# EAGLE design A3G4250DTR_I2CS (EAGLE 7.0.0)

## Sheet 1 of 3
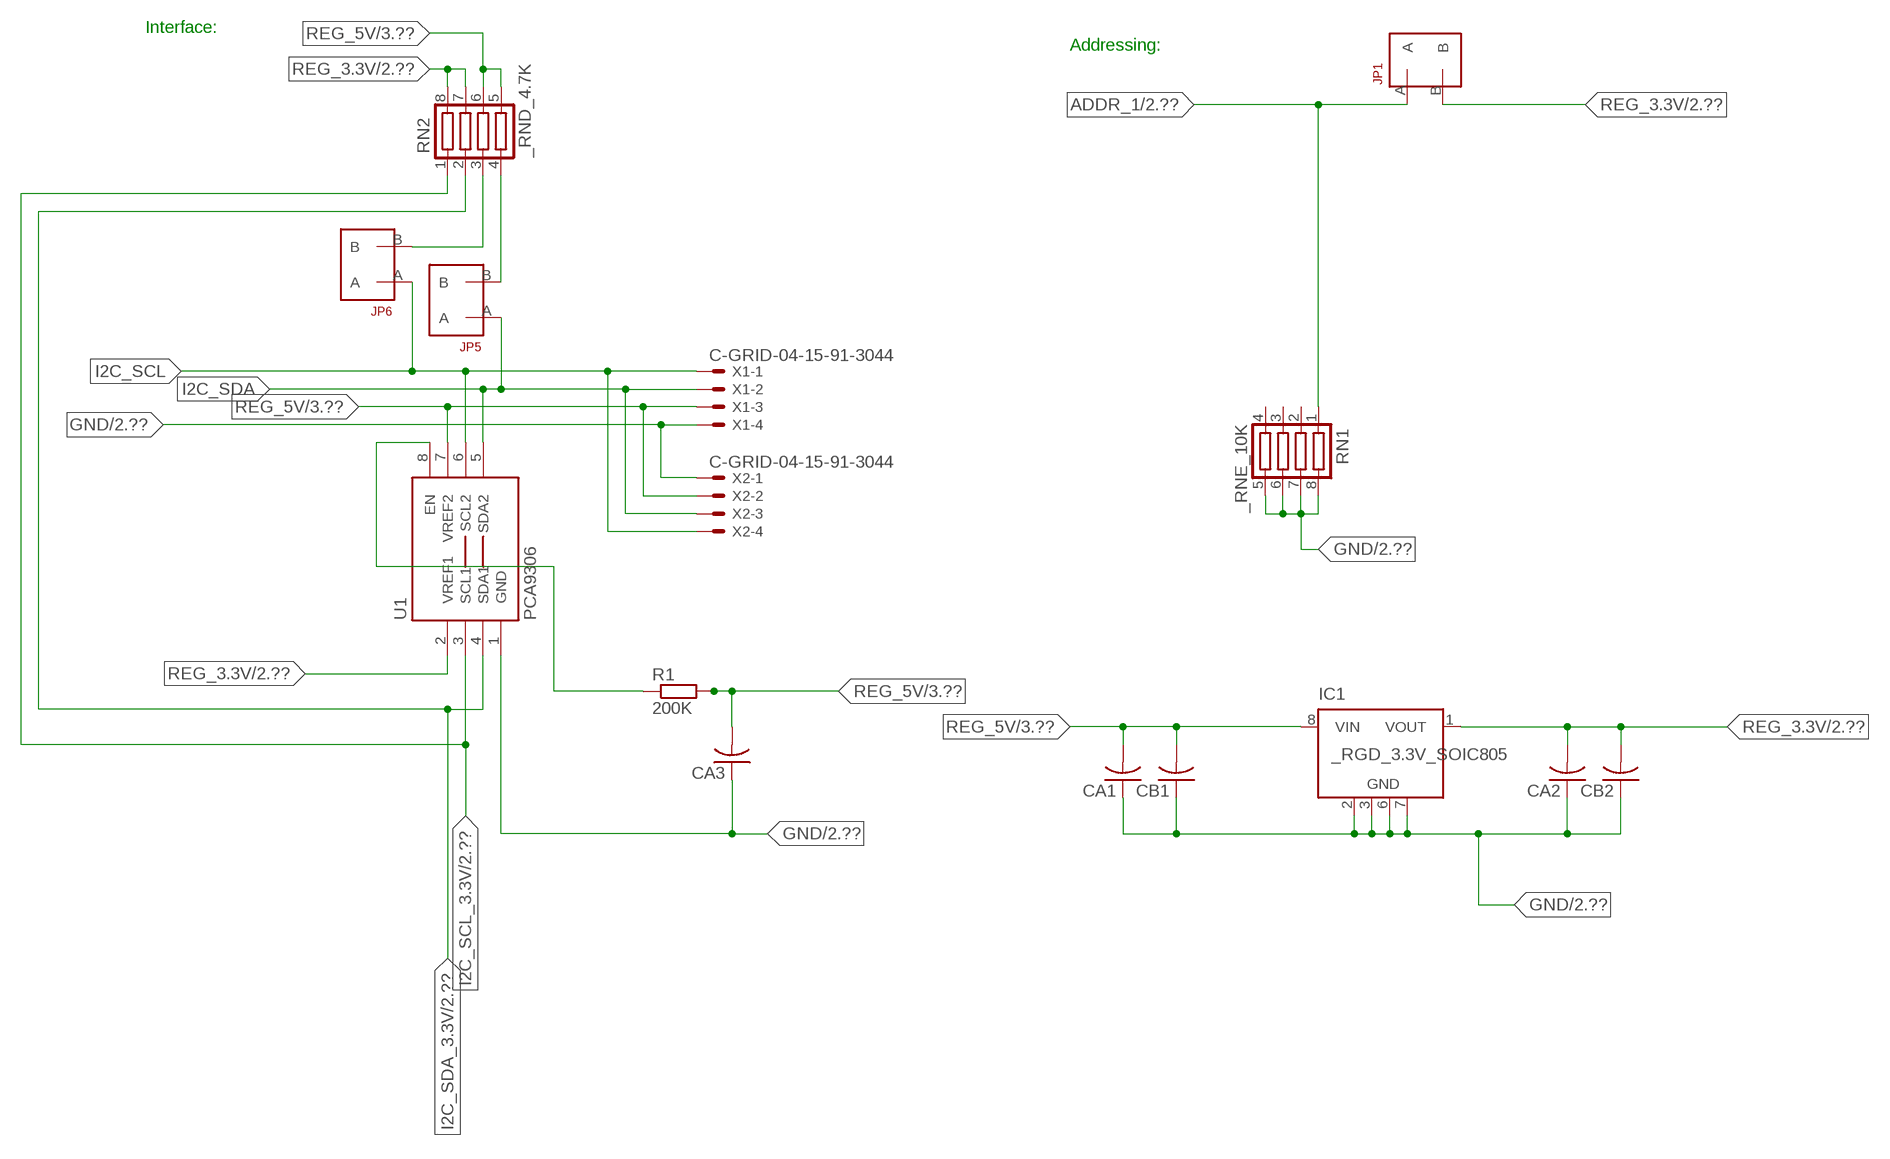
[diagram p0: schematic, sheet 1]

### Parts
CA1  CC1206KRX7R9BB104  [.1UF]
CA2  CC1206KRX7R9BB104  [.1UF]
CA3  CC1206KRX7R9BB104  [.1UF]
CB1  TMK316F106ZL-TC1206K  [TMK316F106ZL-T]
CB2  TMK316F106ZL-TC1206K  [TMK316F106ZL-T]
IC1  _RGD_3.3V_SOIC805  [_RGC_3.3V_SOIC8]
JP1  JUMPER_1X2_2MM  [JUMPER_1X2_2MM]
JP5  JUMPER_1X2_2MM  [JUMPER_1X2_2MM]
JP6  JUMPER_1X2_2MM  [JUMPER_1X2_2MM]
R1  200K  RESISTOR_SMT-0603  [R603]
RN1  _RNE_10K  [RNE]
RN2  _RND_4.7K  [RND]
U1  PCA9306  PCA9306_NCD  [PSOP-8]
X1  C-GRID-04-15-91-3044  [15-91-04]
X2  C-GRID-04-15-91-3044  [15-91-04]

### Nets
ADDR_1: JP1.A RN1.1 ; also sheet 2
GND: CA1.1 CA2.1 CA3.1 CB1.1 CB2.1 IC1.2(GND) IC1.3(GND) IC1.6(GND) IC1.7(GND) RN1.5 RN1.6 RN1.7 RN1.8 U1.1(GND) X1.4 X2.1 ; also sheet 2,3
I2C_SCL: JP6.A U1.6(SCL2) X1.1 X2.4
I2C_SCL_3.3V: RN2.1 U1.3(SCL1) ; also sheet 2
I2C_SDA: JP5.A U1.5(SDA2) X1.2 X2.3
I2C_SDA_3.3V: RN2.2 U1.4(SDA1) ; also sheet 2
N$1: JP6.B RN2.3
N$2: JP5.B RN2.4
N$3: R1.1 U1.8(EN)
REG_3.3V: CA2.2 CB2.2 IC1.1(VOUT) JP1.B RN2.7 RN2.8 U1.2(VREF1) ; also sheet 2
REG_5V: CA1.2 CA3.2 CB1.2 IC1.8(VIN) R1.2 RN2.5 RN2.6 U1.7(VREF2) X1.3 X2.2 ; also sheet 3
Unconnected: IC1.4(NC) IC1.5(NC) RN1.2 RN1.3 RN1.4

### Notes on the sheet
- Interface:
- Addressing:

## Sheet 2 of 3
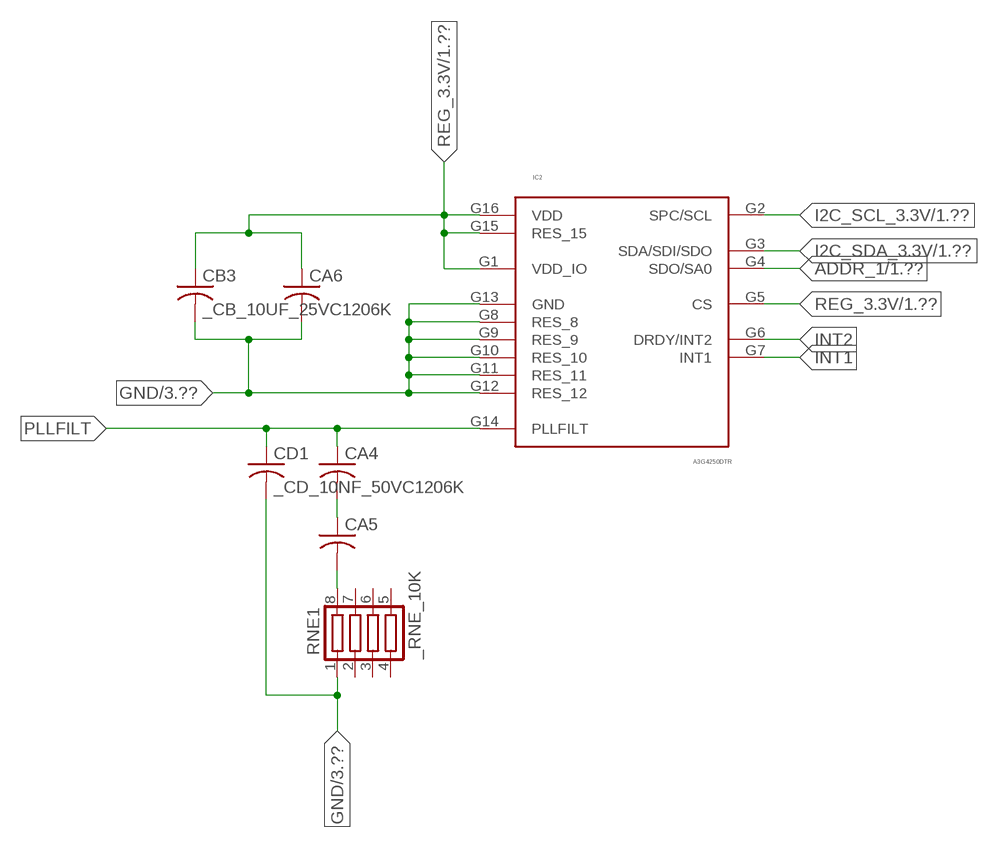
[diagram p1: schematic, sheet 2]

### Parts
CA4  _CA_.10UF_50VC1206K  [_CA_.1UF_50V]
CA5  _CA_.10UF_50VC1206K  [_CA_.1UF_50V]
CA6  _CA_.10UF_50VC1206K  [_CA_.1UF_50V]
CB3  _CB_10UF_25VC1206K  [_CB_10UF_25V]
CD1  _CD_10NF_50VC1206K  [_CD_10NF_50V]
IC2  A3G4250DTR  A3G4250D  [LGA-16]
RNE1  _RNE_10K  [RNE]

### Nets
ADDR_1: IC2.G4(SDO/SA0) ; also sheet 1
GND: CA6.2 CB3.2 CD1.2 IC2.G8(RES_8) IC2.G9(RES_9) IC2.G10(RES_10) IC2.G11(RES_11) IC2.G12(RES_12) IC2.G13(GND) RNE1.1 ; also sheet 1,3
I2C_SCL_3.3V: IC2.G2(SPC/SCL) ; also sheet 1
I2C_SDA_3.3V: IC2.G3(SDA/SDI/SDO) ; also sheet 1
INT1: IC2.G7(INT1)
INT2: IC2.G6(DRDY/INT2)
N$23: CA5.2 RNE1.8
N$24: CA4.2 CA5.1
PLLFILT: CA4.1 CD1.1 IC2.G14(PLLFILT)
REG_3.3V: CA6.1 CB3.1 IC2.G1(VDD_IO) IC2.G5(CS) IC2.G15(RES_15) IC2.G16(VDD) ; also sheet 1
Unconnected: RNE1.2 RNE1.3 RNE1.4 RNE1.5 RNE1.6 RNE1.7

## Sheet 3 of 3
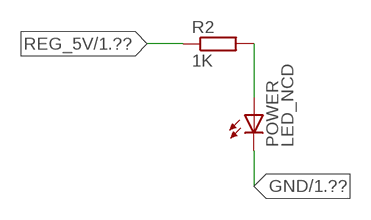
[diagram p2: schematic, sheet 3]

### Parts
POWER  LED_NCD  [CHIPLED_0603]
R2  1K  RESISTOR_SMT-0402  [R402]

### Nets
GND: POWER.C ; also sheet 1,2
N$4: POWER.A R2.2
REG_5V: R2.1 ; also sheet 1

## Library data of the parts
CA1-CA3 = NCD_ULTIMATE_LIBRARY:CC1206KRX7R9BB104: Capacitor CA .1uF 50V SMT C1206K CC1206KRX7R9BB104
CA4-CA6 = NCD_ULTIMATE_LIBRARY (2):_CA_.10UF_50V: Capacitor .1uF SMT
CB1 CB2 = NCD_ULTIMATE_LIBRARY:TMK316F106ZL-T: Capacitor CB 10uF SMT 1206 TMK316F106ZL-T
CB3 = NCD_ULTIMATE_LIBRARY (2):_CB_10UF_25V: Capacitor 10uF SMT
CD1 = NCD_ULTIMATE_LIBRARY (2):_CD_10NF_50V: Capacitor 10nF SMT
IC1 = NCD_ULTIMATE_LIBRARY:_RGD_3.3V_SOIC8: Regulator Linear 3.3V Chip Positive VOLTAGE REGULATOR Digikey 497-1199-2-ND/L78L33ACD13TR
IC2 = NCD_ULTIMATE_KAMNA:A3G4250D
JP1 JP5 JP6 = NCD_ULTIMATE_CONNECTORS:JUMPER_1X2_2MM
POWER = NCD_ULTIMATE_LIBRARY:LED_NCD: LED Digikey 754-1132-2-ND/APT2012SRCPRV
R1 R2 = NCD_ULTIMATE_LIBRARY:RESISTOR_SMT: NCD Resistor
RN1 = NCD_ULTIMATE_LIBRARY:_RNE_10K: Resistor Array RNE SMT 10K x 4 Single Resistor Source: http://www.ctscorp.com/components/Datasheets/CTSChipArrayDs.pdf Digikey 742C083103JPTR-ND/742C083103JP; OC_FARNELL: unknown; OC_NEWARK: unknown
RN2 = NCD_ULTIMATE_LIBRARY:_RND_4.7K: Resistor Array RND SMT 4.7K x 4 Single Resistor Source: http://www.ctscorp.com/components/Datasheets/CTSChipArrayDs.pdf Digikey 742C083472JPTR-ND/742C083472JP; OC_FARNELL: unknown; OC_NEWARK: unknown
RNE1 = NCD_ULTIMATE_LIBRARY (2):_RNE_10K: Resistor Array RNE SMT 10K x 4 Single Resistor Source: http://www.ctscorp.com/components/Datasheets/CTSChipArrayDs.pdf Digikey 742C083103JPTR-ND/742C083103JP; OC_FARNELL: unknown; OC_NEWARK: unknown
U1 = NCD_ULTIMATE_LIBRARY:PCA9306_NCD: NCD Bidirectional I2C level shifter. NOT compatible with all available part number pinout schemes- DOUBLE CHECK!!!; PROD_ID: IC-10023
X1 X2 = NCD_ULTIMATE_CONNECTORS:C-GRID-04: CONNECTOR 4-Pos I2C wire to board 2.54 mm (0.100") pitch header Digikey WM1342-ND/0015912045; OC_FARNELL: unknown; OC_NEWARK: unknown

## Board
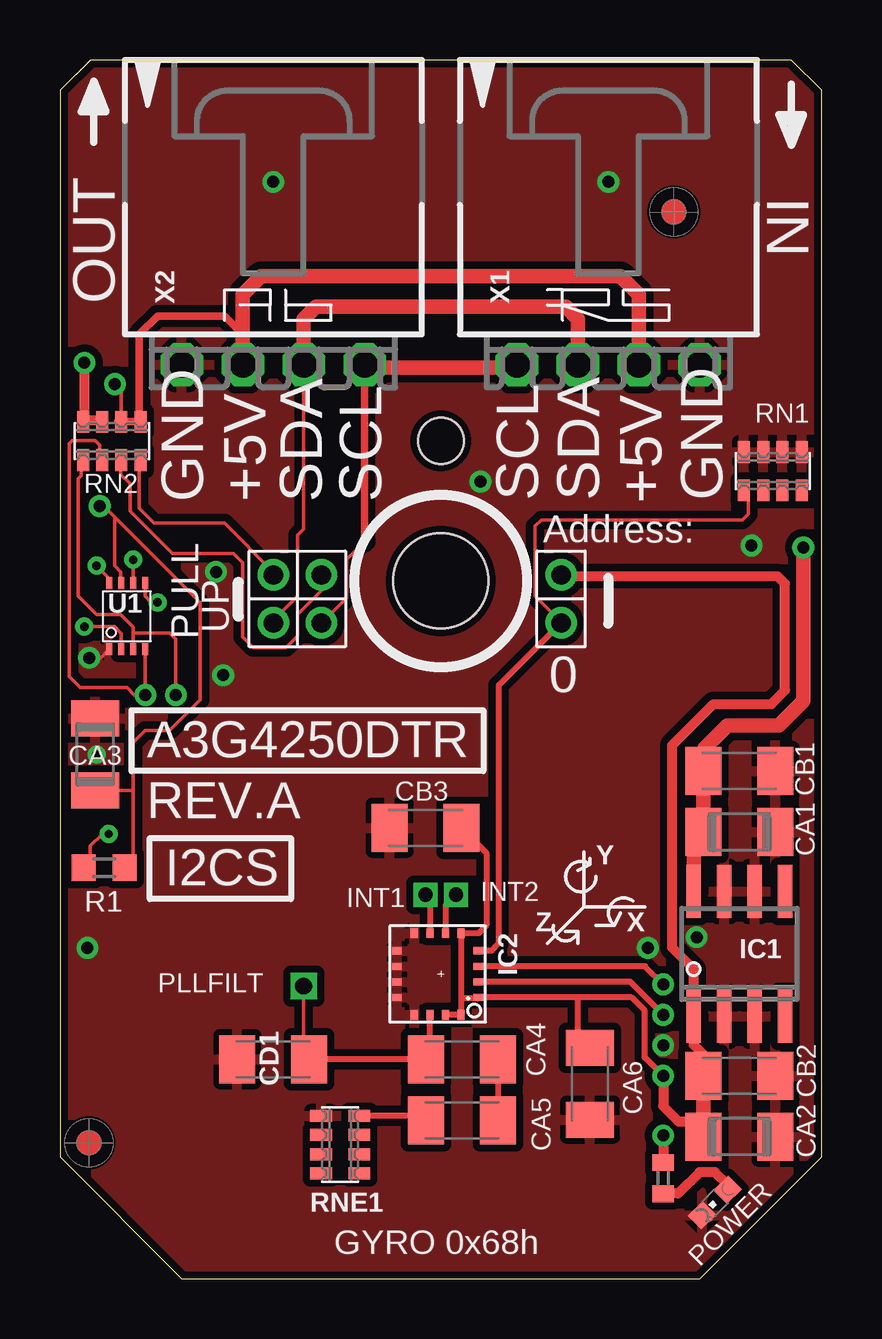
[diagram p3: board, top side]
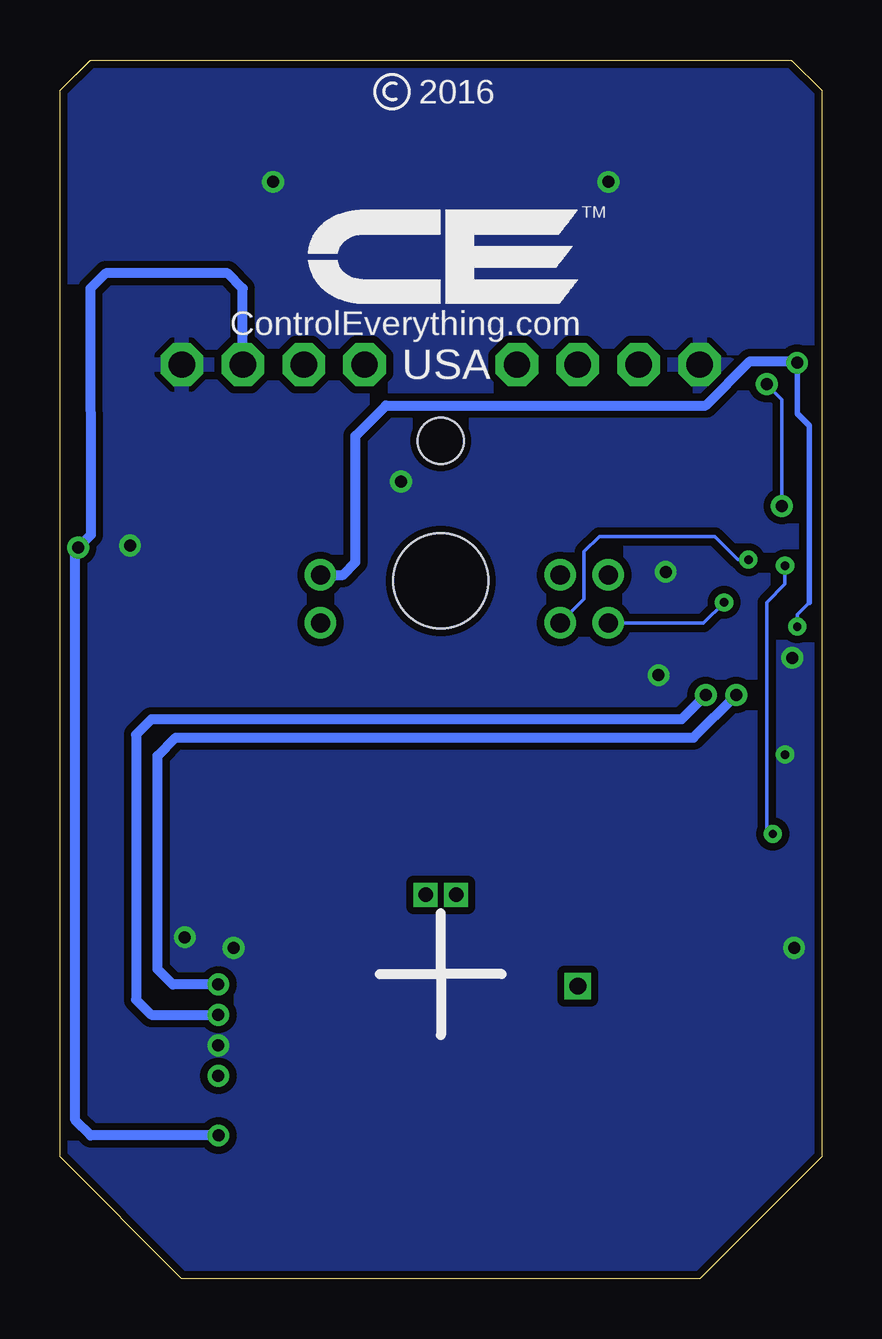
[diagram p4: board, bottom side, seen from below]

Size 31.75 x 50.8 mm. Coordinates in mm from the lower left corner, seen from the top.
Outline: 32 segments
Copper layers (1*16): Top 0.035mm / dielectric 1.5mm / Bottom 0.035mm
Design rules "default": minimum track width 5mil, minimum drill 24mil, track to track 5mil, track to pad 5mil, pad to pad 5mil, via to via 5mil, smd to smd 5mil, copper to edge 10mil, drill to drill 8mil, minimum pad ring 10mil, minimum via ring 8mil, stop-mask expansion 2mil, vias tented up to drill 0mil, thermal gap 10mil
Holes 3.96 mm at 15.88,29.08
Holes 1.91 mm at 15.88,34.93

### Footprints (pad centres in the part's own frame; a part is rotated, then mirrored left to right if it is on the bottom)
.1UF = smd 1.5 x 2: 1 -1.5,0; 2 1.5,0
_CA_.1UF_50V = smd 1.5 x 2: 1 -1.5,0; 2 1.5,0
TMK316F106ZL-T = smd 1.5 x 2: 1 -1.5,0; 2 1.5,0
_CB_10UF_25V = smd 1.5 x 2: 1 -1.5,0; 2 1.5,0
_CD_10NF_50V = smd 1.5 x 2: 1 -1.5,0; 2 1.5,0
_RGC_3.3V_SOIC8 = smd 0.6 x 2.2: 1 -1.905,-2.6; 2 -0.635,-2.6; 3 0.635,-2.6; 4 1.905,-2.6; 5 1.905,2.6; 6 0.635,2.6; 7 -0.635,2.6; 8 -1.905,2.6
LGA-16 = smd 0.4 x 0.3: G1 -1.7,0.975; G2 -1.7,0.325; G3 -1.7,-0.325; G4 -1.7,-0.975; G9 1.7,-0.975; G10 1.7,-0.325; G11 1.7,0.325; G12 1.7,0.975 | smd 0.3 x 0.4: G5 -0.975,-1.7; G6 -0.325,-1.7; G7 0.325,-1.7; G8 0.975,-1.7; G13 0.975,1.7; G14 0.325,1.7; G15 -0.325,1.7; G16 -0.975,1.7
JUMPER_1X2_2MM = drill 0.8: A 0,2; B 0,0
CHIPLED_0603 = smd 0.8 x 0.876: A 0,-0.75; C 0,0.75
R603 = smd 1 x 1.1: 1 -0.85,0; 2 0.85,0
R402 = smd 0.7 x 0.9: 1 -0.65,0; 2 0.65,0
RNE = smd 0.5 x 0.9: 1 -1.2,-0.8; 2 -0.4,-0.8; 3 0.4,-0.8; 4 1.2,-0.8; 5 1.2,0.8; 6 0.4,0.8; 7 -0.4,0.8; 8 -1.2,0.8
RND = smd 0.5 x 0.9: 1 -1.2,-0.8; 2 -0.4,-0.8; 3 0.4,-0.8; 4 1.2,-0.8; 5 1.2,0.8; 6 0.4,0.8; 7 -0.4,0.8; 8 -1.2,0.8
PSOP-8 = smd 0.25 x 0.5: 1 -0.73,-1.37; 2 -0.23,-1.37; 3 0.27,-1.37; 4 0.77,-1.37; 5 0.77,1.38; 6 0.27,1.38; 7 -0.23,1.38; 8 -0.73,1.38
15-91-04 = drill 1.1 pad 1.778 octagon: 1 -3.81,-7.62; 2 -1.27,-7.62; 3 1.27,-7.62; 4 3.81,-7.62

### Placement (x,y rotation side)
CA1  28.32,18.62 180 top
CA2  28.32,5.92 180 top
CA3  1.46,21.86 270 top
CA4  16.76,9.14 0 top
CA5  16.76,6.6 180 top
CA6  22.1,8.13 270 top
CB1  28.32,21.16 180 top
CB2  28.32,8.46 180 top
CB3  15.24,18.8 180 top
CD1  8.89,9.14 180 top
IC1  28.32,13.54 0 top
IC2  15.75,12.7 180 top
JP1  20.89,29.34 180 top
JP5  8.89,29.34 180 top
JP6  10.9,29.34 180 top
POWER  27.3,3.18 135 top
R1  1.84,17.13 0 top
R2  25.15,4.19 270 top
RN1  29.72,33.66 0 top
RN2  2.16,34.93 0 top
RNE1  11.68,5.59 270 top
U1  2.79,27.61 0 top
U$5  [VISION_REF10]  1.21,5.66 90 top
U$28  [VISION_REF10]  25.59,44.46 90 top
X1  22.86,45.72 0 top
X2  8.89,45.72 0 top

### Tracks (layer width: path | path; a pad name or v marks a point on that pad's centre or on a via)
ADDR_1
  Top 0.152: JP1.A 20.89,27.37 19.81,28.45 19.81,31.37 20.07,31.62 28.45,31.62 28.7,31.88 28.7,32.78 RN1.1
  Top 0.254: JP1.A 18.29,24.73 18.29,13.97 17.99,13.68 IC2.G4
GND  (via drill 0.35, 0.5)
  Top 0.152: CA3.1 1.52,23.42 1.52,23.62 | U1.1 1.7,25.88 v1.22,25.88
  other vias: 8.89,45.72 22.86,45.72 25.15,9.73 6.8,25.16 17.53,33.22 26.55,14.24 1.15,13.79 6.5,29.46 1.52,21.84 24.51,13.79 28.83,30.56
  pour Top (isolate 0.305): -1.27,0 -1.27,50.8 33.02,50.8 33.02,0
  pour Bottom (isolate 0.305): -5.08,0 -5.08,50.8 35.56,50.8 35.56,0
I2C_SCL  (via drill 0.35)
  Top 0.152: 12.7,30.73 11.94,29.97 11.94,28.38 JP6.A | v3.05,29.97 3.06,29.96 U1.6
  Top 0.305: 12.7,30.73 X2.4
  Top 0.406: X2.4 12.7,37.97 | 19.05,37.97 X1.1
  Top 0.61: 12.7,37.97 19.05,37.97
  Bottom 0.152: JP6.A 9.91,28.33 9.91,30.3 9.27,30.94 4.45,30.94 3.48,29.97 v3.05,29.97
I2C_SCL_3.3V  (via drill 0.5)
  Top 0.152: RN2.1 0.89,34.07 0.89,33.48 0.77,33.35 0.77,29.1 0.76,29.09 0.76,28.45 1.52,27.69 2.54,27.69 3.06,27.17 3.06,26.92 | 3.06,26.92 U1.3 | v4.83,24.33 v4.83,24.34 4.83,26.67 4.57,26.92 3.06,26.92
  Top 0.254: v25.15,11 23.77,12.38 IC2.G2
  Bottom 0.406: v4.83,24.33 5.84,23.32 27.94,23.32 28.58,22.68 28.58,11.63 27.94,11 v25.15,11
I2C_SDA  (via drill 0.35)
  Top 0.152: JP5.A 8.89,27.44 9.91,28.45 9.91,30.99 10.16,31.24 10.16,34.92 X2.3 | U1.5 3.56,28.45 3.81,28.19 v4.06,28.19
  Top 0.61: X2.3 10.16,40.01 10.67,40.51 21.09,40.51 21.59,40.01 X1.2
  Bottom 0.152: v4.06,28.19 4.92,27.34 JP5.A
I2C_SDA_3.3V  (via drill 0.5)
  Top 0.152: RN2.2 1.65,34.14 1.65,34.75 1.46,34.94 0.51,34.94 0.38,34.81 0.38,26.37 0.38,26.36 0.38,25.1 0.84,24.64 2.79,24.64 3.1,24.33 v3.56,24.33 v3.56,24.34 U1.4
  Top 0.254: v25.15,12.27 24.39,13.03 IC2.G3
  Bottom 0.406: v25.15,12.27 27.05,12.27 27.69,12.9 27.69,21.79 26.93,22.56 5.34,22.56 v3.56,24.33
INT1  (via drill 0.6)
  Top 0.254: v15.24,16 15.42,15.82 IC2.G7
INT2  (via drill 0.6)
  Top 0.254: v16.51,16 16.07,15.57 IC2.G6
N$1
  Top 0.152: JP6.B 10.92,29.31 10.92,28.7 9.91,27.69 9.91,26.8 9.42,26.31 8.06,26.31 7.62,26.75 7.62,29.84 7.24,30.23 4.7,30.23 2.92,32 2.92,33.15 2.54,33.53 2.54,34.1 RN2.3
  Top 0.305: 2.54,34.02 RN2.3
N$2
  Top 0.152: JP5.B 8.89,29.46 6.86,31.5 3.94,31.5 3.3,32.13 3.3,34.07 RN2.4
  Top 0.305: 3.37,33.88 RN2.4
N$3  (via drill 0.35)
  Top 0.152: R1.1 1.27,17.41 1.27,18.03 1.78,18.54 v2.03,18.54 | v1.52,29.72 2.06,29.18 U1.8
  Bottom 0.152: v2.03,18.54 2.29,18.8 2.29,28.19 1.52,28.96 v1.52,29.72
N$4
  Top 0.406: POWER.A 27.84,3.92 27.3,4.45 26.67,4.45 25.78,3.56 25.16,3.56 R2.2
N$23
  Top 0.254: CA5.2 15.08,6.79 RNE1.8
N$24
  Top 0.254: CA4.2 CA5.1
PLLFILT  (via drill 0.7)
  Top 0.152: CD1.1 10.16,9.37 v10.16,12.19
  Top 0.254: IC2.G14 15.42,9.3 CA4.1 CD1.1
REG_3.3V  (via drill 0.35, 0.5)
  Top 0.152: v1.02,27.18 2.29,27.18 2.56,26.9 U1.2
  Top 0.254: 16.72,11.68 IC2.G5 17.45,14.4 17.78,14.73 17.78,17.76 CB3.1 | 16.72,11.68 IC2.G16 IC2.G15 | 16.72,11.68 17.41,11.68 IC2.G1 21.59,11.73 | v25.15,8.46 24.38,9.22 24.38,11.18 23.84,11.73 21.59,11.73 | CA6.1 21.59,10.14 21.59,11.73
  Top 0.406: CB2.2 26.82,9.35 26.42,9.75 26.42,10.36 | v25.15,8.46 25.15,7.19 25.78,6.55 26.82,6.55 | IC1.1 26.42,12.9 25.53,13.79 25.53,22.24 27.24,23.95 29.66,23.95 30.23,24.52 30.23,28.97 29.91,29.29 20.95,29.29 JP1.B | 26.52,5.62 CA2.2 | v1.02,38.18 1.02,35.78 | 1.02,35.78 RN2.8 | 1.02,35.78 1.71,35.78 RN2.7
  Top 0.61: CB2.2 26.82,6.55 CA2.2 | 26.42,10.36 IC1.1
  Bottom 0.152: 0.51,28.19 1.02,27.69 v1.02,27.18
  Bottom 0.229: 0.51,28.19 0.51,35.56 1.02,36.07 v1.02,38.18
  Bottom 0.406: v1.02,38.18 1.08,38.24 2.99,38.24 4.83,36.4 18.16,36.4 19.43,35.13 19.43,29.87 19.94,29.34 JP1.B
REG_5V  (via drill 0.5)
  Top 0.152: RN2.6 2.56,37.01 v2.29,37.29 | R1.2 3.05,17.49 3.05,20.36 | 3.05,20.36 3.05,22.35 3.56,22.86 4.57,22.86 5.84,24.13 5.84,28.19 2.29,31.75 | CA3.2 3.05,20.36 | 2.29,31.75 1.83,32.21 v1.65,32.21 | U1.7 2.54,29.01 2.54,29.46 2.29,29.72 2.29,31.75
  Top 0.305: 7.62,39.37 7.5,39.37 | 2.42,35.74 RN2.6 RN2.5 3.31,35.8 3.31,39.37 4.07,40.13 6.86,40.13 7.62,39.37 | X2.2 7.62,39.37
  Top 0.406: v25.15,5.97 R2.1
  Top 0.61: X1.3 24.13,41.02 23.37,41.78 8.38,41.78 7.62,41.02 X2.2 | IC1.8 26.42,18.21 CA1.2 CB1.2 26.86,21.2 26.86,22.11 27.82,23.06 29.98,23.06 30.99,24.08 v30.99,30.48
  Bottom 0.152: v1.65,32.21 1.65,36.65 v2.29,37.29
  Bottom 0.406: v25.15,5.97 30.48,5.97 31.11,6.6 31.11,30.36 v30.99,30.48 30.47,31 30.48,41.27 29.84,41.91 24.77,41.91 24.13,41.28 24.13,39.37 24.13,38.23 X1.3

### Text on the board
tPlace: Y | Z | X
tNames: IN | OUT | GND | +5V | SDA | SCL | SCL | SDA | +5V | GND | Address: | PULL | UP | 0 | A3G4250DTR | REV.A | I2CS | INT2 | INT1 | PLLFILT | GYRO 0x68h
bNames: 2016 | TM | ControlEverything.com | USA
